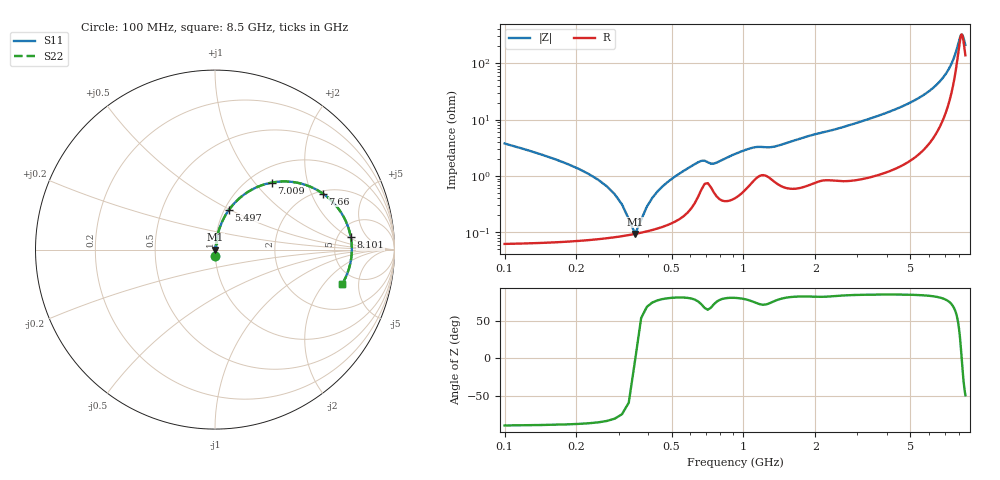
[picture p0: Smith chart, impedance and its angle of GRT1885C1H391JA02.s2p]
!Murata Part Number: GRT1885C1H391JA02
!These Parameters are Measured in Series Mode Connection
!Data Generated on Jun 19, 2026
!  o--ll--o
!Port1  Port2
!  o------o
!Operation Temp=25[degC], DC Bias Voltage=0[V]
!Freq. Start=100[MHz] Stop=9[GHz] 401[Steps]
# Hz S RI R 50
!Freq.(Hz) S11(Real) S11(Imag) S21(Real) S21(Imag) S12(Real) S12(Imag) S22(Real) S22(Imag)
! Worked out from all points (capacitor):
!   401 points, 100 MHz to 8.5 GHz, reference 50 ohm
!   read as one part in series: C = 389 pF near 142 MHz
!   lowest |Z| = 94.1 mohm at 352 MHz (marker M1)
!   series resonance near 352.5 MHz, so ESL is about 520 pH
!   S11 on the Smith chart (normalised r, x): 100 MHz: 1.00, -0.08; 5.497 GHz: 1.05, +0.50; 7.009 GHz: 1.25, +1.23; 7.66 GHz: 2.11, +2.43; 8.101 GHz: 6.57, +2.20; 8.5 GHz: 3.74, -3.14
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1e8  0.00203 -0.0375  0.998 0.0375  0.998 0.0375  0.00203 -0.0375
2.26e8  0.000846 -0.0107  0.9992 0.0107  0.9992 0.0107  0.000846 -0.0107
2.68e8  0.00083 -0.00648  0.9992 0.00648  0.9992 0.00648  0.00083 -0.00648
3.1e8  0.000866 -0.00302  0.9991 0.00302  0.9991 0.00302  0.000866 -0.00302
3.52e8  0.00094 -3.13e-05  0.9991 3.13e-05  0.9991 3.13e-05  0.00094 -3.13e-05
3.94e8  0.00105 0.00265  0.999 -0.00265  0.999 -0.00265  0.00105 0.00265
4.36e8  0.0012 0.00513  0.9988 -0.00513  0.9988 -0.00513  0.0012 0.00513
4.78e8  0.00139 0.00748  0.9986 -0.00748  0.9986 -0.00748  0.00139 0.00748
6.46e8  0.00454 0.0168  0.9955 -0.0168  0.9955 -0.0168  0.00454 0.0168
7.72e8  0.0046 0.0165  0.9954 -0.0165  0.9954 -0.0165  0.0046 0.0165
1.087e9  0.0085 0.0301  0.9915 -0.0301  0.9915 -0.0301  0.0085 0.0301
1.507e9  0.00748 0.0372  0.9925 -0.0372  0.9925 -0.0372  0.00748 0.0372
2.914e9  0.0151 0.0822  0.9849 -0.0822  0.9849 -0.0822  0.0151 0.0822
4.3e9  0.0341 0.1424  0.9659 -0.1424  0.9659 -0.1424  0.0341 0.1424
5.497e9  0.0786 0.2228  0.9214 -0.2228  0.9214 -0.2228  0.0786 0.2228
5.707e9  0.0929 0.2413  0.9071 -0.2413  0.9071 -0.2413  0.0929 0.2413
7.009e9  0.3165 0.3735  0.6835 -0.3735  0.6835 -0.3735  0.3165 0.3735
7.114e9  0.3534 0.3784  0.6466 -0.3784  0.6466 -0.3784  0.3534 0.3784
7.66e9  0.6011 0.312  0.3989 -0.312  0.3989 -0.312  0.6011 0.312
8.101e9  0.7563 0.0708  0.2437 -0.0708  0.2437 -0.0708  0.7563 0.0708
8.248e9  0.7608 -0.0334  0.2392 0.0334  0.2392 0.0334  0.7608 -0.0334
8.5e9  0.7071 -0.1941  0.2929 0.1941  0.2929 0.1941  0.7071 -0.1941
